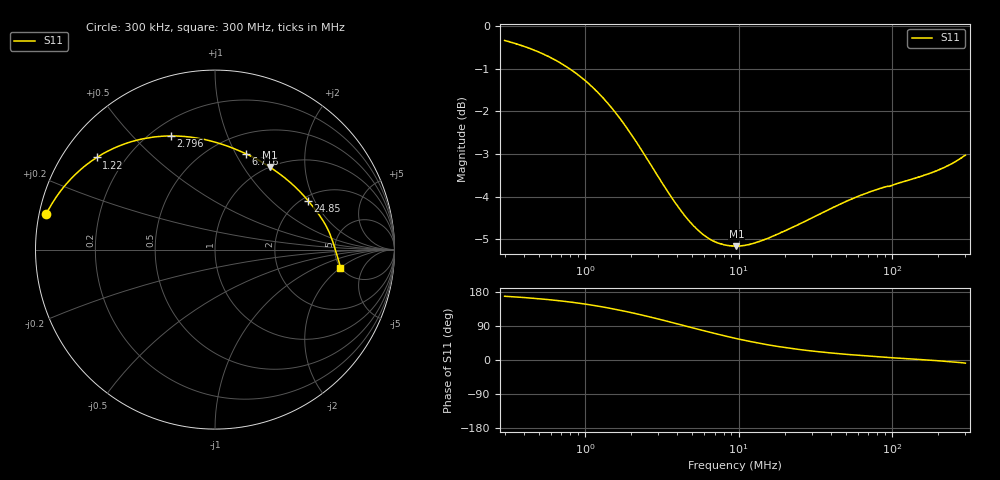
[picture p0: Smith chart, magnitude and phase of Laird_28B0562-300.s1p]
! HEWLETT PACKARD,8753C,0,4.13
! 23 Sep 2019  20:14:37
! frequency  re(S11)  im(S11)
# Hz  S RI R 50
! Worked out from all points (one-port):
!   1601 points, 300 kHz to 300 MHz, reference 50 ohm
!   lowest |S11| = -5.2 dB at 9.694 MHz (marker M1), VSWR 3.46, Z = 50 + j66.2 ohm
!   |S11| at or under -10 dB: nowhere
!   S11 on the Smith chart (normalised r, x): 300 kHz: 0.02, +0.10; 1.22 MHz: 0.10, +0.34; 2.796 MHz: 0.28, +0.65; 6.716 MHz: 0.71, +1.10; 24.85 MHz: 2.15, +1.78; 300 MHz: 4.96, -2.00
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300000  -0.941 0.1966
372281  -0.921 0.2336
476152  -0.8917 0.2818
580759  -0.861 0.3256
714489  -0.8195 0.3755
933782  -0.7498 0.4446
1220382  -0.6581 0.5134
1437956  -0.5899 0.5521
1694321  -0.5137 0.5859
2176437  -0.3838 0.6206
2795733  -0.2468 0.6334
3322736  -0.1528 0.6286
4017871  -0.0543 0.6125
5205897  0.0684 0.5772
6716158  0.1744 0.5331
9527864  0.2989 0.4643
9693837  0.3046 0.4604
1.20815e7  0.369 0.415
1.473569e7  0.4193 0.374
1.797301e7  0.4621 0.3341
2.259412e7  0.5036 0.2899
2.484538e7  0.5186 0.2726
3.570638e7  0.5663 0.2123
5.357913e7  0.6073 0.1519
8.039807e7  0.6365 0.0962
1.27056e8  0.6587 0.0374
2.114684e8  0.6802 -0.0328
3e8  0.6982 -0.1012
